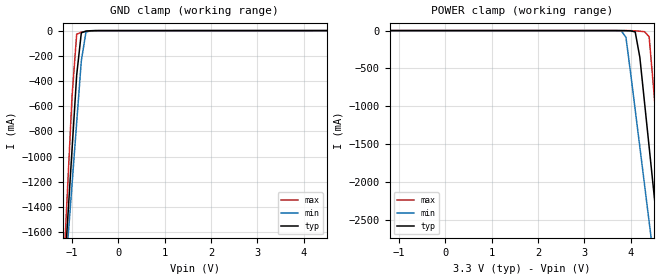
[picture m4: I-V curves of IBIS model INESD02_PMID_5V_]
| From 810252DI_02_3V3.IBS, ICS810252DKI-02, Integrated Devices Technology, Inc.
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[Model]   INESD02_PMID_5V_
Model_type   Input
Polarity   Non-Inverting
Vinl = 0.8V
Vinh = 2.0V
|   typ   min   max
C_comp   2pF   1.5pF   2.5pF
|   typ   min   max
[Voltage range]  3.3V   3.135V   3.465V
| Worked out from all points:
|   GND clamp passes 1 mA (typ) near -0.59 V on its own axis
[GND_clamp]
|Voltage I(typ)   I(min)   I(max)
-3.3V     -14.52A    -12.53A    -17.87A
-1.2V     -2.123A    -2.201A    -2.031A
-1.1V     -1.533A    -1.71A     -1.276A
-1V       -943.1mA   -1.22A     -522.1mA
-900mV    -353.6mA   -729.9mA   -28.78mA
-800mV    -17.87mA   -240.4mA   -12.26mA
-700mV    -3.576mA   -12.1mA    -6.702mA
-600mV    -1.115mA   -934uA     -2.512mA
6.6V      207.5uA    263.8uA    193.2uA
[POWER_clamp]
|Voltage   I(typ)   I(min)   I(max)
-3.3V     128.6uA    156.8uA    124.8uA
3.8V      -180.1uA   -4.403mA   -11.05uA
3.9V      -1.033mA   -88.76mA   -99.86uA
4.1V      -17.79mA   -1.048A    -3.685mA
4.2V      -353.5mA   -1.539A    -8.437mA
4.3V      -943mA     -2.029A    -14.61mA
4.4V      -1.533A    -2.52A     -80.08mA
4.5V      -2.123A    -3.011A    -786mA
4.6V      -2.713A    -3.502A    -1.54A
4.7V      -3.303A    -3.994A    -2.295A
4.8V      -3.894A    -4.485A    -3.049A
6.6V      -14.52A    -13.34A    -16.62A
